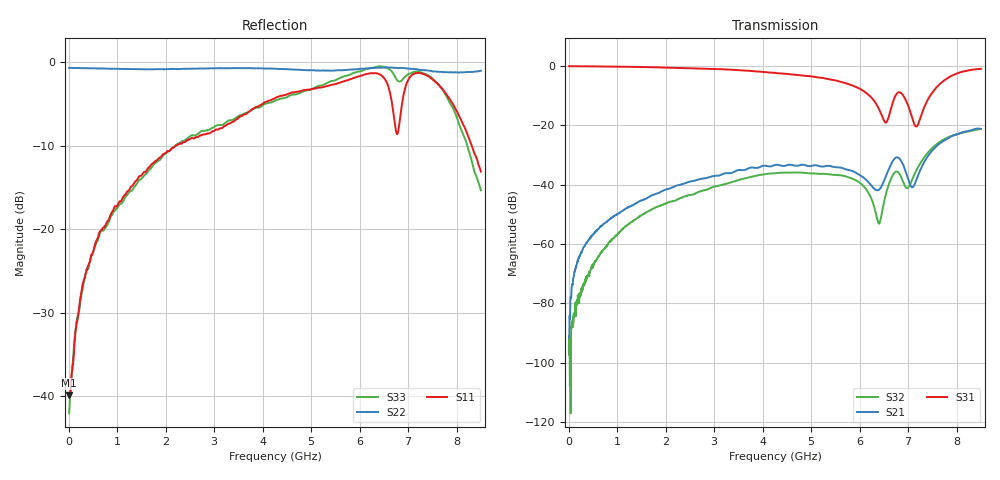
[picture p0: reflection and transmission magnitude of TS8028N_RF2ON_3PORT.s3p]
!Created with skrf (http://scikit-rf.org).
# GHz S RI R 50.0
!freq ReS11 ImS11 ReS12 ImS12 ReS13 ImS13
! ReS21 ImS21 ReS22 ImS22 ReS23 ImS23
! ReS31 ImS31 ReS32 ImS32 ReS33 ImS33
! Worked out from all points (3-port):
!   1601 points, 10 MHz to 8.5 GHz, reference 50 ohm
!   strongest paths, dB at 10 MHz, 2.132 GHz, 4.255 GHz, 6.378 GHz, 8.5 GHz:
!     S31: -0.1, -0.7, -2.4, -13.9, -1.0
!     S21: -91.6, -41.0, -33.4, -41.9, -21.2
!     S32: -97.3, -45.6, -36.1, -52.5, -21.3
!   lowest |S11| = -39.9 dB at 10 MHz (marker M1), VSWR 1.02, Z = 51 - j0.104 ohm
!   |S11| at or under -10 dB: start of sweep to 2.206 GHz; 8.311 GHz to end of sweep
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0.01  0.0101 -0.00102  5.04e-06 2.69e-05  0.9871 -0.00527
      8.33e-06 2.5e-05  -0.9219 0.00491  -3.8e-05 -1.16e-06
      0.9872 -0.0053  8.74e-06 -1.05e-05  0.00787 -0.000781
0.3177625  0.00335 -0.0501  -8.45e-05 0.000892  0.9749 -0.1123
           -7.57e-05 0.000891  -0.9142 0.0908  -0.000162 -0.000131
           0.9751 -0.1124  -0.000171 -0.00011  -0.000996 -0.0487
0.9279812  -0.0298 -0.1282  -0.000633 0.00285  0.9173 -0.3147
           -0.000604 0.00284  -0.8686 0.2753  -0.00126 0.00017
           0.9172 -0.3146  -0.00123 0.000154  -0.0457 -0.1186
4.255  -0.5995 -0.0956  0.00817 0.0198  0.0233 -0.7598
       0.00817 0.0198  -0.2102 0.8877  0.00559 0.0145
       0.021 -0.7607  0.00554 0.0146  -0.582 0.0691
5.884019  -0.6528 0.4696  0.0136 0.0093  -0.3062 -0.3362
          0.0136 0.00927  0.2764 0.8596  0.0115 0.00425
          -0.306 -0.3364  0.0115 0.00424  -0.5058 0.6967
6.398725  -0.4085 0.742  0.00156 0.00807  -0.1453 -0.1188
          0.00151 0.00806  0.3962 0.8353  0.000911 0.00202
          -0.1453 -0.1188  0.000893 0.00202  -0.2216 0.917
6.722406  -0.0909 0.4238  0.00014 0.0275  0.0877 -0.2802
          0.000147 0.0275  0.4393 0.814  -0.0031 0.0157
          0.0877 -0.2804  -0.0031 0.0157  0.0572 0.8209
7.173438  -0.3403 0.7883  -0.00615 0.0105  0.0245 -0.0922
          -0.00609 0.0105  0.4864 0.7644  -0.0114 0.0134
          0.0244 -0.0921  -0.0114 0.0135  0.2583 0.8367
7.773044  0.2473 0.6026  -0.0142 0.0551  0.3635 -0.4657
          -0.0144 0.0552  0.6018 0.6274  0.000115 0.06
          0.3642 -0.4658  6.82e-05 0.0598  0.5651 0.2898
8.5  0.1607 0.1516  0.0412 0.0765  -0.0974 -0.8844
     0.0412 0.0764  0.7683 0.4418  0.0638 0.0583
     -0.0983 -0.8843  0.0638 0.0584  0.1695 -0.021
